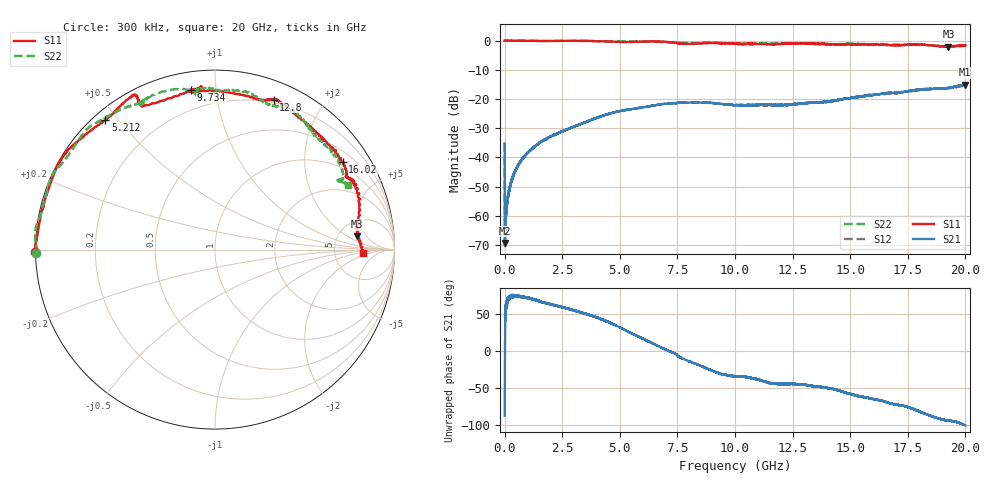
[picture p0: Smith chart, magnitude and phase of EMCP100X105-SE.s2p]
!EMCP100X105
!Johanson Technology Inc.
!www.johansontechnology.com
!Test Board Conditions:
!Substrate Type  RO4350B
!Substrate Thickness  10 mil
!Substrate Dk  3.66
!TL Type: GCPW
!TL Trace Width  20 mil
!TL Gap  10 mil
!PART MODE SINGLE ENDED (AKA BYPASS)
!DUT TOPOLOGY	SERIES-SHUNT
# MHz S  dB  R 50
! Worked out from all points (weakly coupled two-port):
!   20001 points, 300 kHz to 20 GHz, reference 50 ohm
!   highest |S21| = -15.04 dB at 19.99 GHz (marker M1); lowest = -69.4 dB at 15.3 MHz (marker M2)
!   lowest |S11| = -2.0 dB at 19.27 GHz (marker M3), VSWR 8.67, Z = 372 + j150 ohm
!   |S11| at or under -10 dB: nowhere
!   |S22| runs from -2.1 to 0.1 dB; largest |S21 - S12| = 0.0086
!   S11 on the Smith chart (normalised r, x): 300 kHz: -0.00, -0.01; 5.212 GHz: 0.03, +0.46; 9.734 GHz: 0.09, +0.86; 12.8 GHz: 0.17, +1.45; 16.02 GHz: 0.79, +3.04; 20 GHz: 10, -1
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0.3  0.02 -179.3  -35.25 -87.2  -35.20 -87.2  -0.03 -179.0
15.3  0.04 179.9  -69.38 -8.6  -69.41 -6.0  -0.04 179.9
102.298  0.02 179.2  -56.11 63.4  -56.42 62.9  -0.04 179.3
201.297  0.00 178.6  -51.19 74.0  -51.14 72.2  -0.03 178.6
374.294  -0.04 177.1  -46.44 74.9  -46.47 75.1  0.01 177.5
907.286  -0.07 172.2  -39.14 72.9  -39.26 73.2  0.05 173.4
3334.25  -0.06 149.4  -28.45 52.4  -28.51 52.4  -0.06 153.7
5212.222  -0.49 130.3  -23.83 29.1  -23.88 29.5  -0.18 137.8
6667.2  -0.26 117.3  -21.97 7.2  -21.91 6.7  -0.50 125.7
7456.188  -0.72 117.5  -21.39 -3.8  -21.43 -3.8  -0.70 118.0
8745.169  -0.88 95.7  -21.26 -22.8  -21.29 -23.1  -0.71 115.3
9734.154  -0.94 98.6  -21.90 -32.7  -21.80 -31.9  -0.96 98.4
10000.15  -0.98 99.1  -22.12 -33.6  -21.97 -33.2  -1.15 96.1
11548.13  -1.19 74.9  -22.02 -43.1  -22.11 -42.3  -0.91 94.2
12804.11  -0.94 68.6  -21.66 -44.9  -21.58 -45.2  -0.96 82.2
13334.1  -1.01 65.0  -21.29 -47.1  -21.27 -47.4  -1.08 75.7
16017.06  -1.27 34.5  -18.59 -64.8  -18.51 -66.3  -1.30 53.7
16667.05  -1.52 29.4  -17.89 -69.8  -18.18 -69.8  -1.40 50.9
17774.03  -1.39 24.8  -17.17 -78.6  -17.01 -77.8  -1.46 38.2
19266.01  -2.01 5.4  -16.19 -93.7  -16.34 -94.9  -2.12 29.2
19992  -1.64 -1.4  -15.04 -100.2  -15.33 -98.4  -1.67 26.0
20000  -1.65 -1.3  -15.04 -100.4  -15.31 -98.4  -1.67 26.0
